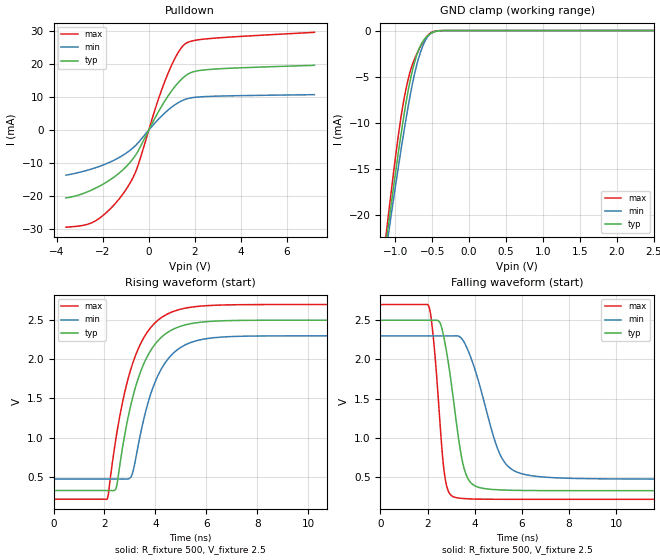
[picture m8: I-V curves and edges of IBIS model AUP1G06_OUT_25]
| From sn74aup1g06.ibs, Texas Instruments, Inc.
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[Model]   AUP1G06_OUT_25
Model_type  Open_drain
Enable   Active-Low
Vref =   2.5
Rref =   1E6
Cref =   30p
Vmeas =   1.25
| variable   typ   min   max
C_comp   1.60pF   1.34pF   1.95pF
| C_pulldown   1.98pF   1.67pF   2.52pF
| C_tri-state   1.60pF   1.34pF   1.95pF
[Temperature Range]   40   100   -40
| Ambient temperature   25   85   -40
[Voltage range]   2.5   2.3   2.7
[Pullup Reference]   2.5   2.5   2.5
[POWER Clamp Reference]   2.5   2.5   2.5
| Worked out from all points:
|   slope of the pulldown table from 0 to 0.375 V, typ, clamps not added: 75.2 ohm
|   GND clamp passes 1 mA (typ) near -0.61 V on its own axis
|   rising waveform, R_fixture 500, V_fixture 2.5: 20-80 % time 1.07ns typ, 1.05ns min, 1.1ns max; typ from 0.325 V to 2.5 V
|   falling waveform, R_fixture 500, V_fixture 2.5: 20-80 % time 615ps typ, 1.06ns min, 384ps max; typ from 2.5 V to 0.325 V
[GND Clamp]
| AUP1G06_OUT_25
|   Voltage   I(typ)   I(min)   I(max)
-3.6V     -193.5mA   -179.7mA   -210.2mA
-1.13V    -23.52mA   -24.27mA   -22.65mA
-1.105V   -21.98mA   -22.86mA   -20.94mA
-1.08V    -20.46mA   -21.47mA   -19.24mA
-935mV    -12.04mA   -13.67mA   -10.14mA
-880mV    -9.138mA   -10.89mA   -7.431mA
-820mV    -6.351mA   -8.054mA   -5.152mA
-745mV    -3.679mA   -4.975mA   -3.233mA
-665mV    -1.77mA    -2.541mA   -1.842mA
-580mV    -733.4uA   -904.6uA   -734uA
-500mV    -240.6uA   -235.7uA   -174.4uA
2.5V      194.1pA    680.1pA    45.53pA
[Pulldown]
| AUP1G06_OUT_25
|   Voltage   I(typ)   I(min)   I(max)
-3.6V     -20.57mA   -13.67mA   -29.41mA
-2.78V    -19.03mA   -12.39mA   -28.76mA
-2.265V   -17.43mA   -11.3mA    -27.29mA
-1.58V    -14.6mA    -9.373mA   -23.19mA
-970mV    -10.98mA   -6.922mA   -17.8mA
-505mV    -6.845mA   -4.179mA   -11.45mA
310mV     4.162mA    2.467mA    7.071mA
775mV     9.655mA    5.67mA     16.13mA
1.215V    13.84mA    8.012mA    22.73mA
1.565V    16.29mA    9.252mA    26.03mA
2.59V     18.34mA    10.19mA    27.69mA
7.2V      19.61mA    10.73mA    29.61mA
[Ramp]
| AUP1G06_OUT_25
| variable   typ   min   max
dV/dt_r   1.31/1.07E-09   1.10/1.05E-09   1.49/1.10E-09
dV/dt_f   1.31/6.16E-10   1.10/1.06E-09   1.49/3.87E-10
R_load = 500
[Rising Waveform]
| AUP1G06_OUT_25
R_fixture =   500
C_fixture =   0
L_fixture =   0
V_fixture =   2.5
V_fixture_min = 2.3
V_fixture_max = 2.7
|   Time   V(typ)   V(min)   V(max)
0s        324.7mV    472mV      214.4mV
2.11ns    324.8mV    472mV      218.4mV
2.465ns   364.8mV    472.1mV    1.019V
3.04ns    1.424V     497.7mV    1.88V
3.24ns    1.669V     757.5mV    2.067V
3.615ns   1.994V     1.332V     2.314V
4.005ns   2.201V     1.724V     2.471V
5.05ns    2.429V     2.163V     2.645V
7.66ns    2.498V     2.296V     2.698V
32.79ns   2.5V       2.3V       2.7V
[Falling Waveform]
| AUP1G06_OUT_25
R_fixture =   500
C_fixture =   0
L_fixture =   0
V_fixture =   2.5
V_fixture_min = 2.3
V_fixture_max = 2.7
|   Time   V(typ)   V(min)   V(max)
0s        2.5V       2.3V       2.7V
2.06ns    2.5V       2.3V       2.672V
2.275ns   2.5V       2.3V       2.188V
2.72ns    2.242V     2.3V       536.9mV
3.19ns    1.274V     2.301V     237.4mV
3.505ns   664.8mV    2.243V     225.1mV
3.85ns    422mV      2.014V     219.6mV
5.08ns    334.8mV    785.7mV    214.9mV
6.19ns    327.2mV    527mV      214.4mV
32.79ns   324.7mV    472mV      214.4mV
